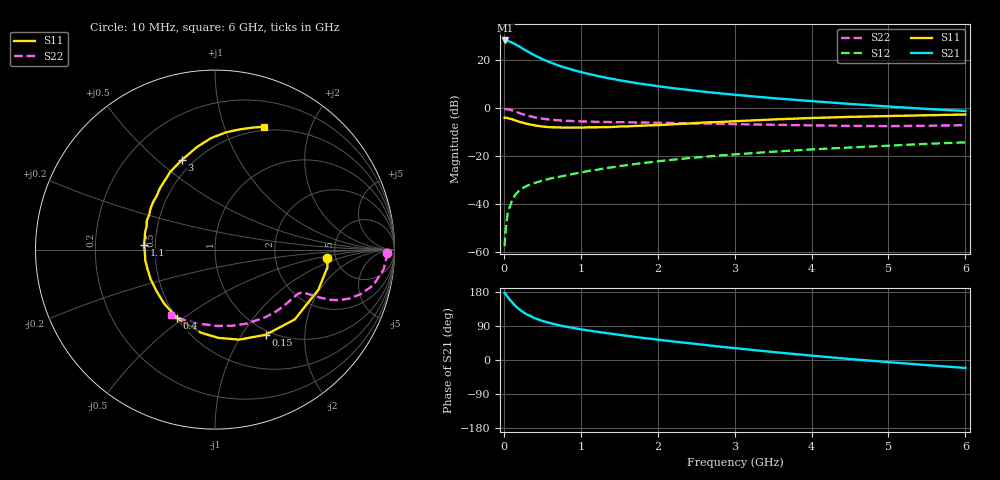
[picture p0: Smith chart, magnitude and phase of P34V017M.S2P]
! SIEMENS Small Signal Semiconductors
! BFP181
! Si NPN RF Bipolar Junction Transistor in SOT143
! VCE = 4 V  IC = 17 mA
! Common Emitter S-Parameters:  March  1996
# GHz  S  MA  R  50
!  f  S11  S21  S12  S22
! GHz  MAG  ANG  MAG  ANG  MAG  ANG  MAG  ANG
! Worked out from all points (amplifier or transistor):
!   36 points, 10 MHz to 6 GHz, reference 50 ohm
!   highest |S21| = 28.3 dB at 20 MHz (marker M1)
!   |S21| within 3 dB of that: start of sweep to 224.1 MHz
!   unconditionally stable (mu >= 1): 739 MHz to end of sweep
!   at 250 MHz: K = 0.50, MSG = 29.1 dB, |S12| = -33.4 dB
!   at 1.4 GHz: K = 1.22, MAG = 15.7 dB, |S12| = -24.8 dB
!   at 6 GHz: K = 1.01, MAG = 6.0 dB, |S12| = -14.3 dB
!   S11 on the Smith chart (normalised r, x): 10 MHz: 4.26, -0.66; 150 MHz: 0.94, -1.28; 400 MHz: 0.50, -0.47; 1.1 GHz: 0.43, +0.03; 3 GHz: 0.43, +0.60; 6 GHz: 0.46, +1.37
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0.01  0.6273 -4.3  25.96 176.9  0.0013 76.4  0.9597 -1.0
0.02  0.6343 -8.9  26 174.5  0.0025 83.4  0.9573 -2.5
0.05  0.6178 -21.2  25.52 166.3  0.0063 85.2  0.9461 -6.7
0.1  0.5906 -41.2  23.67 154.0  0.011 70.6  0.904 -12.7
0.15  0.5521 -59.2  21.6 142.8  0.0155 64.8  0.847 -17.1
0.2  0.5195 -74.9  19.48 133.9  0.019 62.4  0.7908 -20.3
0.25  0.4921 -87.8  17.31 126.4  0.0214 57.8  0.7417 -22.3
0.3  0.4698 -99.5  15.58 120.5  0.0238 55.4  0.7021 -23.5
0.4  0.4357 -119.0  12.72 110.5  0.0273 53.8  0.6411 -24.6
0.5  0.4129 -133.5  10.59 103.3  0.0305 52.7  0.6017 -25.0
0.6  0.3993 -144.6  9.12 97.5  0.0336 52.6  0.5759 -25.5
0.7  0.3947 -155.3  7.878 92.6  0.0362 53.5  0.558 -25.8
0.9  0.393 -170.9  6.29 84.7  0.0422 53.9  0.5357 -26.7
1.1  0.3964 176.3  5.211 77.8  0.0486 54.3  0.5228 -28.3
1.3  0.4015 166.0  4.406 72.0  0.0546 54.5  0.5146 -30.5
1.6  0.4147 152.2  3.607 63.7  0.0641 54.2  0.5055 -33.9
2.2  0.4601 131.7  2.613 48.9  0.0835 51.7  0.489 -42.6
3  0.5318 110.4  1.905 31.4  0.1079 46.2  0.4628 -56.3
3.5  0.5792 100.2  1.617 21.0  0.1226 42.7  0.4495 -66.1
4.5  0.656 84.7  1.224 2.5  0.1504 34.5  0.4258 -88.5
5.5  0.7091 73.3  0.963 -13.5  0.1795 27.2  0.4277 -112.0
6  0.7368 68.3  0.871 -21.0  0.1924 22.7  0.4403 -123.9
